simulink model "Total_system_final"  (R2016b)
settings: Solver=VariableStepAuto  StartTime=0  StopTime=2700  MaxStep=0.1  RelTol=1e-3
undefined symbols (not defined in the file or in its folder): c1, c2, c3, c4, c5, c6, cp_nom, Generation, lambda_nom, P_wind_base, Pelec_base, Pnom, re_lib, speed_nom, Turbine, Wind, wind_base
libraries: simulink x15, simulink_extras x8, dspsigops x7, realtime_pacer_lib x2

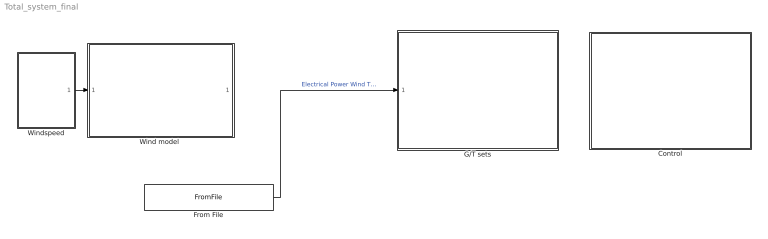
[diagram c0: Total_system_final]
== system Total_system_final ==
  Control : Subsystem
  From File : FromFile  FileName=Pwt_moderate_windtest_6mw_pu  SampleTime=0
  G/T sets : Subsystem
  "Wind model " : Subsystem  Commented=on
  Windspeed : Subsystem
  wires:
  From File/1 -> G/T sets/1(Pe_wind)  "Electrical Power Wind Turbine"
  Windspeed/1(Windspeed) -> "Wind model "/1("windspeed ")

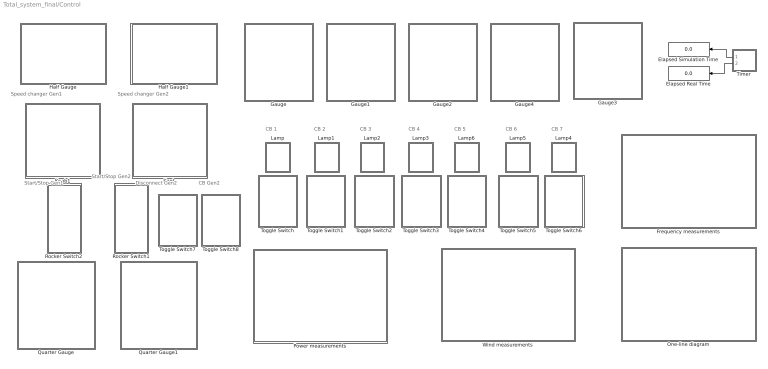
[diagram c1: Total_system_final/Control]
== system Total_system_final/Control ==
  note: Start/Stop Gen1
  note: CB 1
  note: CB 2
  note: CB 3
  note: CB 4
  note: CB 5
  note: CB 6
  note: CB 7
  note: Start/Stop Gen2
  note: Speed changer Gen2
  note: Speed changer Gen1
  note: Disconnect Gen2
  note: CB Gen2
  Elapsed Real Time : Display
  Elapsed Simulation Time : Display
  Frequency measurements : Subsystem
  Gauge : Subsystem  DialogController=hmiCreateDDGDialog  IsWebBlock=on
  Gauge1 : Subsystem  DialogController=hmiCreateDDGDialog  IsWebBlock=on
  Gauge2 : Subsystem  DialogController=hmiCreateDDGDialog  IsWebBlock=on
  Gauge3 : Subsystem  DialogController=hmiCreateDDGDialog  IsWebBlock=on
  Gauge4 : Subsystem  DialogController=hmiCreateDDGDialog  IsWebBlock=on
  Half Gauge : Subsystem  DialogController=hmiCreateDDGDialog  IsWebBlock=on
  Half Gauge1 : Subsystem  DialogController=hmiCreateDDGDialog  IsWebBlock=on
  Knob : Subsystem  DialogController=hmiCreateDDGDialog  IsWebBlock=on
  Knob1 : Subsystem  DialogController=hmiCreateDDGDialog  IsWebBlock=on
  Lamp : Subsystem  Tag=CB1  DialogController=hmiCreateDDGDialog  IsWebBlock=on
  Lamp1 : Subsystem  DialogController=hmiCreateDDGDialog  IsWebBlock=on
  Lamp2 : Subsystem  DialogController=hmiCreateDDGDialog  IsWebBlock=on
  Lamp3 : Subsystem  DialogController=hmiCreateDDGDialog  IsWebBlock=on
  Lamp4 : Subsystem  DialogController=hmiCreateDDGDialog  IsWebBlock=on
  Lamp5 : Subsystem  DialogController=hmiCreateDDGDialog  IsWebBlock=on
  Lamp6 : Subsystem  DialogController=hmiCreateDDGDialog  IsWebBlock=on
  One-line diagram : Subsystem
  Power measurements : Subsystem
  Quarter Gauge : Subsystem  DialogController=hmiCreateDDGDialog  IsWebBlock=on
  Quarter Gauge1 : Subsystem  DialogController=hmiCreateDDGDialog  IsWebBlock=on
  Rocker Switch1 : Subsystem  DialogController=hmiCreateDDGDialog  IsWebBlock=on
  Rocker Switch2 : Subsystem  DialogController=hmiCreateDDGDialog  IsWebBlock=on
  Timer : Subsystem
  Toggle Switch : Subsystem  DialogController=hmiCreateDDGDialog  IsWebBlock=on
  Toggle Switch1 : Subsystem  DialogController=hmiCreateDDGDialog  IsWebBlock=on
  Toggle Switch2 : Subsystem  DialogController=hmiCreateDDGDialog  IsWebBlock=on
  Toggle Switch3 : Subsystem  DialogController=hmiCreateDDGDialog  IsWebBlock=on
  Toggle Switch4 : Subsystem  DialogController=hmiCreateDDGDialog  IsWebBlock=on
  Toggle Switch5 : Subsystem  DialogController=hmiCreateDDGDialog  IsWebBlock=on
  Toggle Switch6 : Subsystem  DialogController=hmiCreateDDGDialog  IsWebBlock=on
  Toggle Switch7 : Subsystem  DialogController=hmiCreateDDGDialog  IsWebBlock=on
  Toggle Switch8 : Subsystem  DialogController=hmiCreateDDGDialog  IsWebBlock=on
  Wind measurements : Subsystem
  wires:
  Timer/2(Out2) -> Elapsed Real Time/1
  Timer/1(Out1) -> Elapsed Simulation Time/1

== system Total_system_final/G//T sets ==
  Pe_wind : Inport
  G/T sets : Subsystem
  Load : Subsystem
  Load shedding : Subsystem
  Mux : Mux  Inputs=2
  Scope : Scope
  Scope1 : Scope
  Start & Stop : Subsystem
  Switches : Subsystem
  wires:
  Mux/1 -> Scope/1
  G/T sets/1(Gen1freq) -> Scope1/1, Mux/1  "Frequency Gen 1"
  G/T sets/2(Gen2Freq) -> Mux/2  "Frequency Gen 2"
  Pe_wind/1 -> Load/1(Pe_wind)
  Load/1(Pe_Gen) -> Start & Stop/1(Pe_Gen), G/T sets/2(Last)
  Switches/2(Disc_Gen_2) -> G/T sets/6(Disc)
  Switches/3(Auto) -> G/T sets/1(auto), Start & Stop/3(Auto)
  Switches/6(StartStopp_Gen1) -> Start & Stop/4(StartStop_Gen1)
  Switches/7(StartStopp_Gen2) -> Start & Stop/5(StartStop_Gen2)
  Switches/4(SpeedChanger1) -> G/T sets/4(speedchanger1)
  Switches/5(SpeedChanger2) -> G/T sets/5(speedchanger2)
  Switches/1(CB_Man) -> G/T sets/3(CB_man), Start & Stop/2(CB_man)

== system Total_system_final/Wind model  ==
  "windspeed " : Inport
  Drive train model : Subsystem
  Mux : Mux  Inputs=2
  Pitch : Subsystem
  Scope : Scope
  Scope1 : Scope
  To File : ToFile  Commented=on  Filename=Pwt_moderate_windtest_6MW.mat  MatrixName=Pwt_moderate_windtest_6MW  SaveFormat=Timeseries
  Wind Turbine : Subsystem  AncestorBlock=re_lib/Wind Generation/Wind Turbine  DialogController=POWERSYS.PowerSysDialog
  Pe : Outport
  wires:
  Drive train model/1(w) -> Scope/1, Wind Turbine/1(Generator speed (pu))
  Wind Turbine/1(Tm (pu)) -> Pitch/1(Tm), Drive train model/1(Tm), Mux/1
  "windspeed "/1 -> Wind Turbine/3(Wind speed (m/s)), Pitch/2(windspeed)
  Pitch/1(ß) -> Wind Turbine/2(Pitch angle (deg))
  Mux/1 -> Scope1/1
  Drive train model/2(Pe_ref) -> To File/1, Pe/1, Mux/2

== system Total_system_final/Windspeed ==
  From File1 : FromFile  FileName=wind_forecast2.mat  SampleTime=0
  From File3 : FromFile  FileName=windserie_test.mat  SampleTime=0
  Mux : Mux  Inputs=2
  Scope : Scope
  Scope1 : Scope
  Scope2 : Scope
  Windspeed : Outport
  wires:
  From File1/1 -> Mux/1, Scope/1  "Wind forecast"
  From File3/1 -> Mux/2, Scope1/1, Windspeed/1  "Wind speed m/s"
  Mux/1 -> Scope2/1

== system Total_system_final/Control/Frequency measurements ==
  Dashboard Scope : Subsystem  DialogController=hmiCreateDDGDialog  IsWebBlock=on
  Dashboard Scope1 : Subsystem  DialogController=hmiCreateDDGDialog  IsWebBlock=on

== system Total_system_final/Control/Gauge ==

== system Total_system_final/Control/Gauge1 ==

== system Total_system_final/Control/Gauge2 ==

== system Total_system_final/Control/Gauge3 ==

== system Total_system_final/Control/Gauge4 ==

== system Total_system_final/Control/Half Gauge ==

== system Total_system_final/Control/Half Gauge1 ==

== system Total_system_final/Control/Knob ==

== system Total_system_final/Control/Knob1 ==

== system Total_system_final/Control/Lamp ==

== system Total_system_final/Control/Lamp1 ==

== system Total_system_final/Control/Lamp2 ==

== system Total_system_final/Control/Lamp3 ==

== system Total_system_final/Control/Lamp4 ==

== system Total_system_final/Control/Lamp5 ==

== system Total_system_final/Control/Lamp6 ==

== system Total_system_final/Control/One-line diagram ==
  MultiStateImage : Subsystem  DialogController=hmiCreateDDGDialog  IsWebBlock=on

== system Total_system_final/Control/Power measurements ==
  Dashboard Scope : Subsystem  DialogController=hmiCreateDDGDialog  IsWebBlock=on
  Dashboard Scope1 : Subsystem  DialogController=hmiCreateDDGDialog  IsWebBlock=on
  Dashboard Scope2 : Subsystem  DialogController=hmiCreateDDGDialog  IsWebBlock=on
  Dashboard Scope3 : Subsystem  DialogController=hmiCreateDDGDialog  IsWebBlock=on

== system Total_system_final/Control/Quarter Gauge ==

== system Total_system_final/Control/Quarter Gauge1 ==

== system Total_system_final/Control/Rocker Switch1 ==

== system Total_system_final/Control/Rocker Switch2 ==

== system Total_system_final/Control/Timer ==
  Clock : Clock
  Elapsed Real Time1 : realtime_pacer_lib/Elapsed Real Time
  Real-Time Pacer : realtime_pacer_lib/Real-Time Pacer  simTimePerRealTime=15
  Scope5 : Scope
  Subtract : Sum  Inputs=+-
  Out1 : Outport
  Out2 : Outport  Port=2
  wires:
  Clock/1 -> Out1/1, Subtract/1
  Subtract/1 -> Scope5/1  "Simulated - Real Time (seconds)"
  Elapsed Real Time1/1 -> Out2/1, Subtract/2

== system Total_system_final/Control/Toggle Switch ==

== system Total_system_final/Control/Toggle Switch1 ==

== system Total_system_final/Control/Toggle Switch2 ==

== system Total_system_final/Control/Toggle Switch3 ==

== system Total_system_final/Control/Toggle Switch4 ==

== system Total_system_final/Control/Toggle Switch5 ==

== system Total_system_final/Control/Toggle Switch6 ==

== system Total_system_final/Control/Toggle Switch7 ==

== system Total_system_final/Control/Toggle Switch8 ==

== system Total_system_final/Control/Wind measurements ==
  Dashboard Scope : Subsystem  DialogController=hmiCreateDDGDialog  IsWebBlock=on
  Dashboard Scope1 : Subsystem  DialogController=hmiCreateDDGDialog  IsWebBlock=on

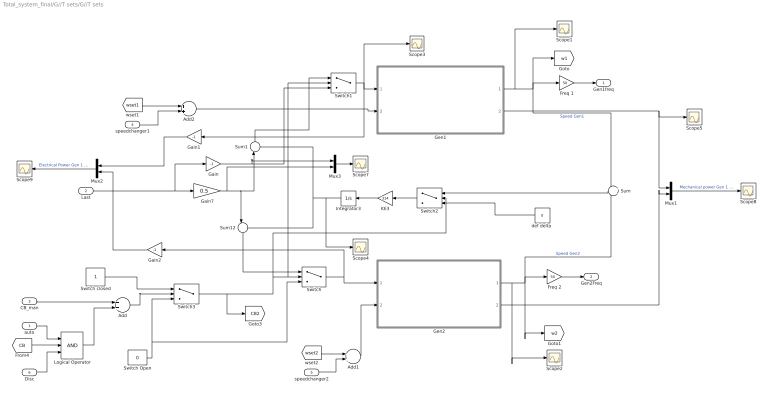
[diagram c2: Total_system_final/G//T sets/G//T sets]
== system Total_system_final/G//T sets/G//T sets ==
  auto : Inport
  Last : Inport  Port=2
  CB_man : Inport  Port=3
  speedchanger1 : Inport  Port=4
  speedchanger2 : Inport  Port=5
  Disc : Inport  Port=6
  Add : Sum
  Add1 : Sum
  Add2 : Sum
  Freq 1 : Gain  Gain=50
  Freq 2 : Gain  Gain=50
  Gain : Gain  Gain=-1
  Gain1 : Gain  Gain=-1
  Gain2 : Gain  Gain=-1
  Gain7 : Gain  Gain=0.5
  Gen1 : Subsystem
  Gen2 : Subsystem
  Integrator3 : Integrator  UpperSaturationLimit=0.0001  LowerSaturationLimit=-0.0001
  KE3 : Gain  Gain=314
  Logical Operator : Logic  Inputs=3  AllPortsSameDT=off  OutDataTypeStr=boolean
  Mux1 : Mux  Inputs=2
  Mux2 : Mux  Inputs=2
  Mux3 : Mux  Inputs=2
  Scope{1..5,7..9} (8 alike) : Scope
  Sum : Sum  Inputs=+-
  Sum1 : Sum  Inputs=--
  Sum12 : Sum  Inputs=|-+
  Switch{,1..3} (4 alike) : Switch  Criteria=u2 > Threshold
  Switch Open : Constant  Value=0
  Switch closed : Constant
  "def delta " : Constant  Value=0
  Gen1freq : Outport
  Gen2Freq : Outport  Port=2
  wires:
  Gen2/1(w2) -> Scope2/1, [w2], Sum/2, Freq 2/1  "Speed Gen2"
  Gen1/1(w1) -> Scope1/1, [w1], Sum/1, Freq 1/1  "Speed Gen1"
  Mux1/1 -> Scope8/1  "Mechanical power Gen 1 and 2"
  Gen1/2(Pm1) -> Scope5/1, Mux1/1
  Gen2/2(Pm2) -> Mux1/2
  Mux2/1 -> Scope9/1  "Electrical Power Gen 1 & 2"
  Gain7/1 -> Mux3/2, Sum1/1, Sum12/1
  Switch2/1 -> KE3/1
  Switch1/1 -> Scope3/1, Gain1/1, Gen1/1(Pe)
  Sum1/1 -> Switch1/1
  Switch/1 -> Gen2/1(Pe), Gain2/1
  Sum12/1 -> Switch/1
  Switch3/1 -> [CB2], Switch2/2, Switch1/2, Switch/2
  Switch Open/1 -> Switch/3, Switch3/3
  Switch closed/1 -> Switch3/1
  Gain/1 -> Mux3/1, Switch1/3
  Integrator3/1 -> Scope4/1, Sum1/2, Sum12/2
  KE3/1 -> Integrator3/1
  "def delta "/1 -> Switch2/3
  Freq 1/1 -> Gen1freq/1
  Freq 2/1 -> Gen2Freq/1
  Mux3/1 -> Scope7/1
  speedchanger1/1 -> Add2/2
  [wset1] -> Add2/1
  Add2/1 -> Gen1/2(wset1)
  Add/1 -> Switch3/2
  Last/1 -> Gain/1, Gain7/1
  Add1/1 -> Gen2/2(wset2)
  speedchanger2/1 -> Add1/2
  Logical Operator/1 -> Add/2
  [CB] -> Logical Operator/2
  auto/1 -> Logical Operator/1
  CB_man/1 -> Add/1
  Disc/1 -> Logical Operator/3
  Gain1/1 -> Mux2/1
  Gain2/1 -> Mux2/2
  Sum/1 -> Switch2/1
  [wset2] -> Add1/1

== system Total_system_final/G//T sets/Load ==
  Pe_wind : Inport
  Add : Sum  Inputs=+-
  Local base --> System base : Gain  Gain=6/13
  Pe_Gen : Outport
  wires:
  Add/1 -> Pe_Gen/1
  Local base --> System base/1 -> Add/2, [P_wind]  "Electrical Power Wind turbine"
  [Pe_load] -> Add/1  "Electrical load"
  Pe_wind/1 -> Local base --> System base/1

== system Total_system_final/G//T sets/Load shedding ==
  Display{,1..3,5..8} (8 alike) : Display
  Load shedding : Subsystem
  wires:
  Load shedding/2(Open CB_B1M1) -> Display/1
  Load shedding/1(∆Pe_G1) -> [Pe_load]
  Load shedding/3(Open CB_B1M2) -> Display1/1
  Load shedding/4(Open CB_B1L1) -> Display2/1
  Load shedding/5(Open CB_B1M3) -> Display3/1
  [w1] -> Load shedding/1(w_G1)
  Load shedding/7(Open CB_B1B4) -> Display6/1
  Load shedding/6(Open CB_B1M4) -> Display5/1
  Load shedding/8(Open CB_B4B5) -> Display7/1
  Load shedding/9(idx) -> Display8/1

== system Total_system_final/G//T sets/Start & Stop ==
  Pe_Gen : Inport
  CB_man : Inport  Port=2
  Auto : Inport  Port=3
  StartStop_Gen1 : Inport  Port=4
  StartStop_Gen2 : Inport  Port=5
  StartStop : MATLAB Function  TreatAsAtomicUnit=on
  TransportDelay : TransportDelay  DelayTime=400
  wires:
  Pe_Gen/1 -> StartStop/1(P_Gen)
  CB_man/1 -> StartStop/2(CB_man)
  Auto/1 -> StartStop/7(auto)
  StartStop/2(wset2) -> [wset2]
  StartStop/3(CB_auto) -> TransportDelay/1
  [w2] -> StartStop/4(w2)
  TransportDelay/1 -> StartStop/8(Connect), [CB]
  [w1] -> StartStop/3(w1)
  StartStop/1(wset1) -> [wset1]
  StartStop_Gen1/1 -> StartStop/5(start_stop_G1)
  StartStop_Gen2/1 -> StartStop/6(start_stop_G2)

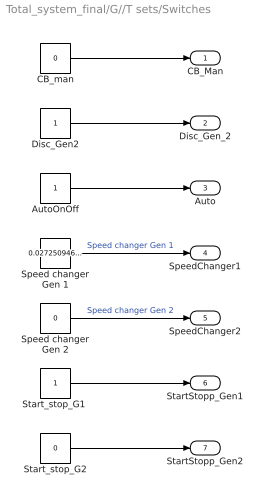
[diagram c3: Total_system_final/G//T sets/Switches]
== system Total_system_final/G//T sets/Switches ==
  AutoOnOff : Constant
  CB_man : Constant  Value=0
  Disc_Gen2 : Constant
  Speed changer Gen 1 : Constant  Value=0.0272509460449
  Speed changer Gen 2 : Constant  Value=0
  "Start_stop_G1 " : Constant
  Start_stop_G2 : Constant  Value=0
  CB_Man : Outport
  Disc_Gen_2 : Outport  Port=2
  Auto : Outport  Port=3
  SpeedChanger1 : Outport  Port=4
  SpeedChanger2 : Outport  Port=5
  StartStopp_Gen1 : Outport  Port=6
  StartStopp_Gen2 : Outport  Port=7
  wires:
  "Start_stop_G1 "/1 -> StartStopp_Gen1/1
  AutoOnOff/1 -> Auto/1
  Disc_Gen2/1 -> Disc_Gen_2/1
  CB_man/1 -> CB_Man/1
  Speed changer Gen 1/1 -> SpeedChanger1/1  "Speed changer Gen 1"
  Speed changer Gen 2/1 -> SpeedChanger2/1  "Speed changer Gen 2"
  Start_stop_G2/1 -> StartStopp_Gen2/1

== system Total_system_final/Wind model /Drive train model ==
  Tm : Inport
  Controller : Subsystem
  Gain : Gain  Gain=1/(2*5)
  Integrator : Integrator  InitialCondition=1  LimitOutput=on  UpperSaturationLimit=2  LowerSaturationLimit=0
  Sum : Sum  Inputs=|+|-
  Transfer Fcn : TransferFcn  Denominator=[2 1]
  w : Outport
  Pe_ref : Outport  Port=2
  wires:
  Tm/1 -> Sum/1
  Sum/1 -> Gain/1
  Gain/1 -> Integrator/1
  Integrator/1 -> Controller/1(In1), w/1
  Transfer Fcn/1 -> Pe_ref/1, Sum/2
  Controller/1(Out1) -> Transfer Fcn/1

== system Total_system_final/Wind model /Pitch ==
  Tm : Inport
  windspeed : Inport  Port=2
  Delay : TransferFcn  Denominator=[0.1 1]
  Integrator Limited : Integrator  LimitOutput=on  UpperSaturationLimit=90  LowerSaturationLimit=0
  PI : Subsystem
  Rate Limiter : RateLimiter  RisingSlewLimit=5  FallingSlewLimit=-5
  Saturation2 : Saturate  UpperLimit=90  LowerLimit=0  ZeroCross=off
  Saturation3 : Saturate  UpperLimit=1  LowerLimit=-1  ZeroCross=off
  Sum1 : Sum  Inputs=|+|-
  Sum2 : Sum  Inputs=|+-
  Tm_ref : Constant
  ß : Outport
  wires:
  Tm_ref/1 -> Sum1/2
  Delay/1 -> Rate Limiter/1
  Rate Limiter/1 -> Integrator Limited/1
  windspeed/1 -> PI/2(Wind speed)
  Saturation3/1 -> PI/1(∆Tm)
  PI/1(Out1) -> Saturation2/1
  Sum2/1 -> Delay/1
  Saturation2/1 -> Sum2/1
  Sum1/1 -> Saturation3/1
  Tm/1 -> Sum1/1
  Integrator Limited/1 -> Sum2/2, ß/1

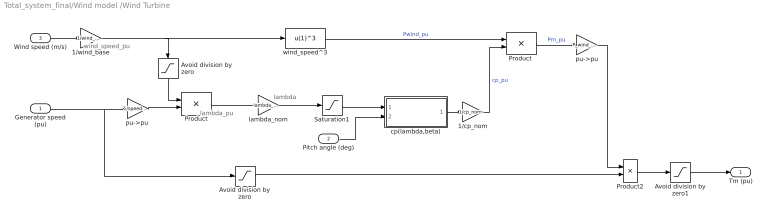
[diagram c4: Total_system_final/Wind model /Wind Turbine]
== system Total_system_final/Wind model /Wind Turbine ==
  note: wind_speed_pu
  note: lambda_pu
  note: lambda
  Generator speed (pu) : Inport
  Pitch angle (deg) : Inport  Port=2
  Wind speed (m/s) : Inport  Port=3
  1/cp_nom : Gain  Gain=1/cp_nom
  1/wind_base : Gain  Gain=1/wind_base
  Avoid division by zero : Saturate  UpperLimit=1e6  LowerLimit=1e-6
  "Avoid division by zero " : Saturate  UpperLimit=1e6  LowerLimit=1e-6
  Avoid division by zero1 : Saturate  UpperLimit=3  LowerLimit=0
  Product : Product  Inputs=/*
  "Product " : Product
  Product2 : Product  Inputs=*/
  Saturation1 : Saturate  UpperLimit=inf  LowerLimit=1e-6
  cp(lambda,beta) : Subsystem
  lambda_nom : Gain  Gain=lambda_nom
  pu->pu : Gain  Gain=P_wind_base*Pnom/Pelec_base
  "pu->pu " : Gain  Gain=1/speed_nom
  wind_speed^3 : Fcn  Expr=u(1)^3
  Tm (pu) : Outport
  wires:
  Pitch angle (deg)/1 -> cp(lambda,beta)/2(beta)
  pu->pu/1 -> Product2/1
  cp(lambda,beta)/1(cp) -> 1/cp_nom/1
  wind_speed^3/1 -> "Product "/1  "Pwind_pu"
  Avoid division by zero/1 -> Product2/2
  Wind speed (m/s)/1 -> 1/wind_base/1
  Generator speed (pu)/1 -> Avoid division by zero/1, "pu->pu "/1
  "Product "/1 -> pu->pu/1  "Pm_pu"
  lambda_nom/1 -> Saturation1/1
  1/cp_nom/1 -> "Product "/2  "cp_pu"
  Saturation1/1 -> cp(lambda,beta)/1(lambda)
  Product/1 -> lambda_nom/1
  1/wind_base/1 -> wind_speed^3/1, "Avoid division by zero "/1
  "Avoid division by zero "/1 -> Product/1
  "pu->pu "/1 -> Product/2
  Product2/1 -> Avoid division by zero1/1
  Avoid division by zero1/1 -> Tm (pu)/1

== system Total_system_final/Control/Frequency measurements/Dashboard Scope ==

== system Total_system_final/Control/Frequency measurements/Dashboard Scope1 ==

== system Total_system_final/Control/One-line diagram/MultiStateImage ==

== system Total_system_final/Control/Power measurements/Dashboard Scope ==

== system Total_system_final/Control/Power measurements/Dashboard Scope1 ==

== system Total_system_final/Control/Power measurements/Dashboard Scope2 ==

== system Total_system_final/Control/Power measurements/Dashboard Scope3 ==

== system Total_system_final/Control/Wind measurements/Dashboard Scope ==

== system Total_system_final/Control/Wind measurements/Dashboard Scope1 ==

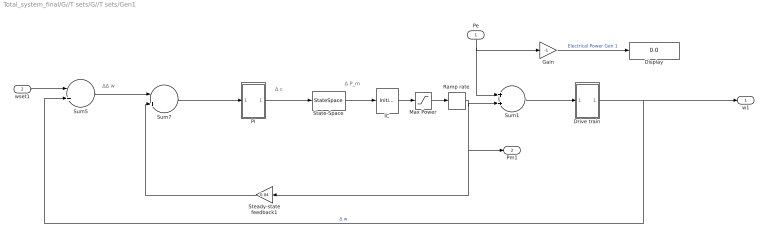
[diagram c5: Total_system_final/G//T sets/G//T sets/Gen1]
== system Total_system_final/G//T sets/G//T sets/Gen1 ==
  note: ∆∆ w
  note: ∆ c
  note: ∆ P_m
  Pe : Inport
  wset1 : Inport  Port=2
  Display : Display
  Drive train : Subsystem
  Gain : Gain  Gain=-1
  IC : InitialCondition
  Max Power : Saturate  Commented=through  UpperLimit=1.2  LowerLimit=-0.2
  PI : Subsystem
  Ramp rate : RateLimiter  Commented=through  RisingSlewLimit=0.05  SampleTimeMode=inherited
  State-Space : StateSpace  A=-5  C=5  D=0  X0=0
  Steady-state feedback1 : Gain  Gain=0.04
  Sum1 : Sum
  Sum5 : Sum  Inputs=|+|-
  Sum7 : Sum  Inputs=|+|-
  w1 : Outport
  Pm1 : Outport  Port=2
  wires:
  Pe/1 -> Sum1/1, Gain/1
  Sum5/1 -> Sum7/1
  Steady-state feedback1/1 -> Sum7/2
  Sum7/1 -> PI/1(In1)
  Sum1/1 -> Drive train/1(In1)
  wset1/1 -> Sum5/1
  Drive train/1(Out1) -> w1/1, Sum5/2  "∆ w"
  PI/1(Out1) -> State-Space/1
  Gain/1 -> Display/1  "Electrical Power Gen 1"
  Max Power/1 -> Ramp rate/1
  Ramp rate/1 -> Steady-state feedback1/1, Pm1/1, Sum1/2
  State-Space/1 -> IC/1
  IC/1 -> Max Power/1

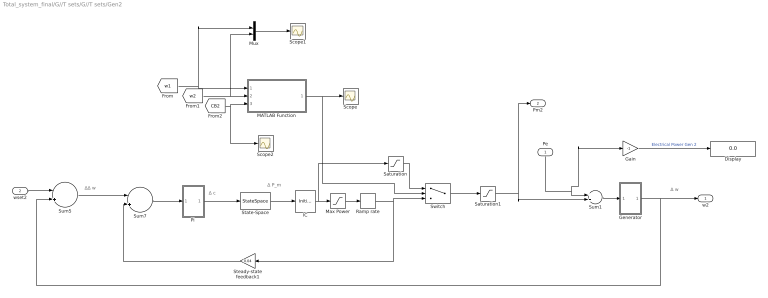
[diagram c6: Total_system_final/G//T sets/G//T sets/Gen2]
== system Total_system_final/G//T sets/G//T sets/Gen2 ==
  note: ∆∆ w
  note: ∆ w
  note: ∆ c
  note: ∆ P_m
  Pe : Inport
  wset2 : Inport  Port=2
  Display : Display
  Gain : Gain  Gain=-1
  Generator : Subsystem
  IC : InitialCondition  Commented=through
  MATLAB Function : MATLAB Function  TreatAsAtomicUnit=on
  Max Power : Saturate  Commented=through  UpperLimit=1.05  LowerLimit=-0.2
  Mux : Mux  Inputs=2
  Pi : Subsystem
  Ramp rate : RateLimiter  Commented=through  RisingSlewLimit=0.038  SampleTimeMode=inherited
  Saturation : Saturate  UpperLimit=0.05  LowerLimit=-0.1  LinearizeAsGain=off
  Saturation1 : Saturate  UpperLimit=1.05  LowerLimit=-0.2
  Scope : Scope
  Scope1 : Scope
  Scope2 : Scope
  State-Space : StateSpace  A=-5  C=5  D=0  X0=0
  Steady-state feedback1 : Gain  Gain=0.04
  Sum1 : Sum
  Sum5 : Sum  Inputs=|+|-
  Sum7 : Sum  Inputs=|+|-
  Switch : Switch  Criteria=u2 > Threshold
  w2 : Outport
  Pm2 : Outport  Port=2
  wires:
  Sum5/1 -> Sum7/1
  Steady-state feedback1/1 -> Sum7/2
  wset2/1 -> Sum5/1
  Sum1/1 -> Generator/1(In1)
  Generator/1(Out1) -> w2/1, Sum5/2
  Sum7/1 -> Pi/1(In1)
  [w1] -> Mux/1, MATLAB Function/1(w1)
  [w2] -> Mux/2, MATLAB Function/2(w2)
  Pi/1(Out1) -> State-Space/1
  Saturation/1 -> Switch/1
  MATLAB Function/1(x) -> Switch/2, Scope/1
  [CB2] -> Scope2/1, MATLAB Function/3(CB)
  Pe/1 -> Gain/1, Sum1/1
  Gain/1 -> Display/1  "Electrical Power Gen 2"
  Mux/1 -> Scope1/1
  Saturation1/1 -> Sum1/2, Pm2/1
  Switch/1 -> Saturation1/1
  Max Power/1 -> Ramp rate/1
  IC/1 -> Saturation/1, Max Power/1
  State-Space/1 -> IC/1
  Ramp rate/1 -> Steady-state feedback1/1, Switch/3

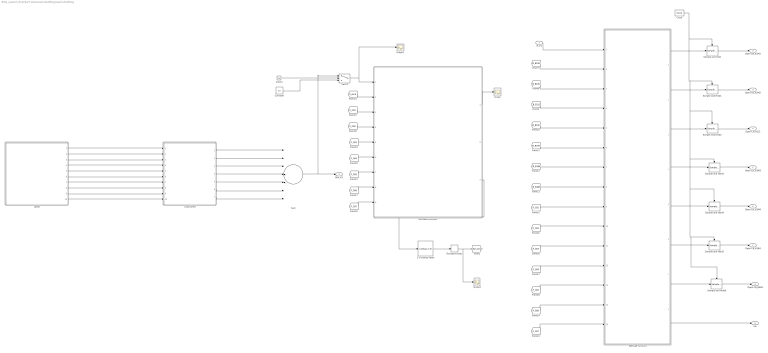
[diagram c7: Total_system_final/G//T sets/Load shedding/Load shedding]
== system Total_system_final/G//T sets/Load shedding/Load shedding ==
  w_G1 : Inport
  1-D Lookup Table : Lookup_n-D  NumberOfTableDimensions=1  BreakpointsForDimension1=[0,1,2,3,4,5,6,7]  Table=[0 10, 12, 14, 16, 18, 20, 22]  InternalRulePriority=Speed  RndMeth=Simplest
  Clock : simulink_extras/Flip Flops/Clock  period=10
  Clock1 : Clock
  Constant : Constant  Value=0.8
  Load_Shed : Subsystem
  Loads : Subsystem
  MATLAB Function : MATLAB Function  TreatAsAtomicUnit=on
  MATLAB Function1 : MATLAB Function  TreatAsAtomicUnit=on
  Sample and Hold{,1..6} (7 alike) : dspsigops/Sample and Hold  trig=Rising edge  initCond=0  latchinput=off
  Scope : Scope
  Scope1 : Scope
  Scope2 : Scope
  Sum : Sum  Inputs=+++++++
  Switch : Switch  Criteria=u2 > Threshold  Threshold=199
  Transport Delay : TransportDelay
  ∆Pe_G1 : Outport
  Open CB_B1M1 : Outport  Port=2
  Open CB_B1M2 : Outport  Port=3
  Open CB_B1L1 : Outport  Port=4
  Open CB_B1M3 : Outport  Port=5
  Open CB_B1M4 : Outport  Port=6
  Open CB_B1B4 : Outport  Port=7
  Open CB_B4B5 : Outport  Port=8
  idx : Outport  Port=9
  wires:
  w_G1/1 -> MATLAB Function/1(freq)
  Loads/1("Load M1 ") -> Load_Shed/1(" Load M1")
  Loads/10(Load M7) -> Load_Shed/10(Load M7)
  Loads/9(Load L3) -> Load_Shed/9(Load L3)
  Loads/8(Load M6) -> Load_Shed/8(Load M6)
  Loads/7(Load M5) -> Load_Shed/7(Load M5)
  Loads/6(Load L2) -> Load_Shed/6(Load L2)
  Loads/5(Load M4) -> Load_Shed/5(Load M4)
  Loads/4(Load M3) -> Load_Shed/4(Load M3)
  Loads/3(Load L1) -> Load_Shed/3(Load L1)
  Loads/2(Load M2) -> Load_Shed/2(Load M2)
  [CB_B1M1] -> MATLAB Function/2(CB_B1M1)
  [CB_B1M2] -> MATLAB Function/3(CB_B1M2)
  [CB_B1L1] -> MATLAB Function/4(CB_B1L1)
  [CB_B1M3] -> MATLAB Function/5(CB_B1M3)
  [CB_B1M4] -> MATLAB Function/6(CB_B1M4)
  [CB_B1B4] -> MATLAB Function/7(CB_B1B4)
  [CB_B4B5] -> MATLAB Function/8(CB_B4B5)
  [P_CB1] -> MATLAB Function/9(P_CB_B1M1)
  [P_CB2] -> MATLAB Function/10(P_CB_B1M2)
  [P_CB3] -> MATLAB Function/11(P_CB_B1L1)
  [P_CB4] -> MATLAB Function/12(P_CB_B1M3)
  [P_CB5] -> MATLAB Function/13(P_CB_B1M4)
  [P_CB6] -> MATLAB Function/14(P_CB_B1B4)
  [P_CB7] -> MATLAB Function/15(P_CB_B4B5)
  MATLAB Function/1(CB_B1M1_stat) -> Sample and Hold/1
  Sample and Hold/1 -> Open CB_B1M1/1
  MATLAB Function/8(idx) -> idx/1
  MATLAB Function/2(CB_B1M2_stat) -> Sample and Hold1/1
  Sample and Hold1/1 -> Open CB_B1M2/1
  Sample and Hold2/1 -> Open CB_B1L1/1
  MATLAB Function/3(CB_B1L1_stat) -> Sample and Hold2/1
  Sample and Hold3/1 -> Open CB_B1M3/1
  MATLAB Function/4(CB_B1M3_stat) -> Sample and Hold3/1
  Sample and Hold4/1 -> Open CB_B1M4/1
  MATLAB Function/5(CB_B1M4_stat) -> Sample and Hold4/1
  MATLAB Function/6(CB_B1B4_stat) -> Sample and Hold5/1
  Sample and Hold5/1 -> Open CB_B1B4/1
  MATLAB Function/7(CB_B4B5_stat) -> Sample and Hold6/1
  Sample and Hold6/1 -> Open CB_B4B5/1
  Clock/1 -> Sample and Hold6/Trigger, Sample and Hold5/Trigger, Sample and Hold4/Trigger, Sample and Hold3/Trigger, Sample and Hold2/Trigger, Sample and Hold1/Trigger, Sample and Hold/Trigger
  Sum/1 -> Switch/1, ∆Pe_G1/1
  [P_wind] -> MATLAB Function1/2(P_wind)
  MATLAB Function1/1(Power) -> Scope/1
  [P_CB1] -> MATLAB Function1/3(P_CB_B1M1)
  [P_CB2] -> MATLAB Function1/4(P_CB_B1M2)
  [P_CB3] -> MATLAB Function1/5(P_CB_B1L1)
  [P_CB4] -> MATLAB Function1/6(P_CB_B1M3)
  [P_CB5] -> MATLAB Function1/7(P_CB_B1M4)
  [P_CB6] -> MATLAB Function1/8(P_CB_B1B4)
  [P_CB7] -> MATLAB Function1/9(P_CB_B4B5)
  MATLAB Function1/3(CB) -> 1-D Lookup Table/1
  1-D Lookup Table/1 -> Transport Delay/1
  Transport Delay/1 -> [CB2_auto2], Scope2/1
  Load_Shed/1(Power_CB_B1M1) -> Sum/1
  Load_Shed/2(Power_CB_B1M2) -> Sum/2
  Load_Shed/3(Power_CB_B1L1) -> Sum/3
  Load_Shed/4(Power_CB_B1M3) -> Sum/4
  Load_Shed/5(Power_CB_B1M4) -> Sum/5
  Load_Shed/6(Power_CB_B4B5) -> Sum/6
  Load_Shed/7(Power_CB_B1B4) -> Sum/7
  Switch/1 -> Scope1/1, MATLAB Function1/1(P_load)
  Clock1/1 -> Switch/2
  Constant/1 -> Switch/3

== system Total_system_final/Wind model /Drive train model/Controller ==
  In1 : Inport
  Fcn : Fcn  Expr=u^2
  "MW -> pu" : Gain  Gain=1/(6e6)
  Product : Product
  Subsystem : Subsystem
  "pu -> rad/sec" : Gain  Gain=11*((2*3.14)/60)
  Out1 : Outport
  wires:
  Product/1 -> "MW -> pu"/1
  Fcn/1 -> Product/1
  Subsystem/1(K-opt) -> Product/2
  "pu -> rad/sec"/1 -> Fcn/1
  In1/1 -> "pu -> rad/sec"/1
  "MW -> pu"/1 -> Out1/1

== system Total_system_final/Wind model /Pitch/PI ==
  ∆Tm : Inport
  Wind speed : Inport  Port=2
  Gain scheduling : Lookup_n-D  NumberOfTableDimensions=1  BreakpointsForDimension1=[10,12,14,15,16,17,18,19,20,21,22,23,24,25]  Table=[20,20,20,20,20,20,20,20,15,15,15,15,15,15]  InternalRulePriority=Speed  RndMeth=Simplest
  Integral constant : Constant  Value=3.11111
  PI Controller : simulink/Continuous/PID Controller  Controller=PI  TimeDomain=Continuous-time  SampleTime=-1  IntegratorMethod=Forward Euler  FilterMethod=Forward Euler  Form=Parallel  UseFilter=on  ControllerParametersSource=external  P=1  I=1  D=0  N=100  InitialConditionSource=internal  InitialConditionForIntegrator=0  InitialConditionForFilter=0  ExternalReset=none  LimitOutput=on  UpperSaturationLimit=90  LowerSaturationLimit=0  LinearizeAsGain=on  AntiWindupMode=clamping  Kb=1  TrackingMode=off  Kt=1  PParamMin=[]  PParamMax=[]  IParamMin=[]  IParamMax=[]  DParamMin=[]  DParamMax=[]  NParamMin=[]  NParamMax=[]  KbParamMin=[]  KbParamMax=[]  KtParamMin=[]  KtParamMax=[]  POutMin=[]  POutMax=[]  IOutMin=[0]  IOutMax=[]  DOutMin=[]  DOutMax=[]  NOutMin=[]  NOutMax=[]  KbOutMin=[]  KbOutMax=[]  KtOutMin=[]  KtOutMax=[]  IntegratorOutMin=[]  IntegratorOutMax=[]  FilterOutMin=[]  FilterOutMax=[]  SumOutMin=[]  SumOutMax=[]  SumI1OutMin=[]  SumI1OutMax=[]  SumI2OutMin=[]  SumI2OutMax=[]  SumI3OutMin=[]  SumI3OutMax=[]  SumDOutMin=[]  SumDOutMax=[]  SaturationOutMin=[]  SaturationOutMax=[]  IntegratorContinuousStateAttributes=''  IntegratorStateMustResolveToSignalObject=off  IntegratorRTWStateStorageClass=Auto  FilterContinuousStateAttributes=''  FilterStateMustResolveToSignalObject=off  FilterRTWStateStorageClass=Auto  DifferentiatorICPrevScaledInput=0  DifferentiatorOutMin=[]  DifferentiatorOutMax=[]
  Out1 : Outport
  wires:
  Gain scheduling/1 -> PI Controller/2
  Wind speed/1 -> Gain scheduling/1
  ∆Tm/1 -> PI Controller/1
  PI Controller/1 -> Out1/1
  Integral constant/1 -> PI Controller/3

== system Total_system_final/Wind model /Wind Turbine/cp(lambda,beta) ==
  lambda : Inport
  beta : Inport  Port=2
  Fcn : Fcn  Expr=1/(1/(u[1]+0.08*u[2])-0.035/(u[2]^3+1))
  Fcn1 : Fcn  Expr=c1*(c2/u[2]-c3*u[3]-c4)*exp(-c5/u[2])+c6*u[1]
  Mux : Mux  Inputs=2
  Mux1 : Mux  Inputs=3
  Scope1 : Scope
  Scope2 : Scope  NumInputPorts=2
  Scope3 : Scope
  cp : Outport
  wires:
  Fcn/1 -> Scope1/1, Mux1/2  "lambda_i"
  Fcn1/1 -> Scope3/1, cp/1
  lambda/1 -> Scope2/1, Mux1/1, Mux/1
  Mux1/1 -> Fcn1/1
  beta/1 -> Scope2/2, Mux1/3, Mux/2
  Mux/1 -> Fcn/1

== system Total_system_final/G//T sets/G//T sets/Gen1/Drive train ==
  In1 : Inport
  " D" : Gain  Gain=0
  Gain4 : Gain  Gain=1/(2*5)
  Integrator Limited1 : Integrator  InitialCondition=1  UpperSaturationLimit=2  LowerSaturationLimit=0
  Sum8 : Sum  Inputs=+-
  Out1 : Outport
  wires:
  Sum8/1 -> Gain4/1
  Gain4/1 -> Integrator Limited1/1
  In1/1 -> Sum8/1
  " D"/1 -> Sum8/2
  Integrator Limited1/1 -> " D"/1, Out1/1

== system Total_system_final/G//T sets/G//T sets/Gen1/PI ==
  In1 : Inport
  Derivative : Derivative
  Gain1 : Gain  Gain=0.8
  Gain3 : Gain  Gain=5
  Gain5 : Gain  Gain=1.2
  Integrator1 : Integrator  InitialCondition=0.5
  Sum6 : Sum  Inputs=|+|+|+
  Out1 : Outport
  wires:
  Sum6/1 -> Out1/1
  Integrator1/1 -> Sum6/2
  Gain5/1 -> Integrator1/1
  In1/1 -> Gain1/1, Gain5/1, Gain3/1
  Gain3/1 -> Sum6/1
  Gain1/1 -> Derivative/1
  Derivative/1 -> Sum6/3

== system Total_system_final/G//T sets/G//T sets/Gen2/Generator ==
  In1 : Inport
  " D" : Gain  Gain=0
  Gain4 : Gain  Gain=1/(2*5)
  Integrator Limited1 : Integrator  UpperSaturationLimit=2  LowerSaturationLimit=0
  Sum8 : Sum  Inputs=+-
  Out1 : Outport
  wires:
  Sum8/1 -> Gain4/1
  Gain4/1 -> Integrator Limited1/1
  In1/1 -> Sum8/1
  " D"/1 -> Sum8/2
  Integrator Limited1/1 -> " D"/1, Out1/1

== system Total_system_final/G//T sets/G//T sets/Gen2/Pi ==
  In1 : Inport
  Derivative : Derivative
  Gain1 : Gain  Gain=0.8
  Gain3 : Gain  Gain=5
  Gain5 : Gain  Gain=1.2
  Integrator1 : Integrator  InitialCondition=0.5
  Sum6 : Sum  Inputs=|+|+|+
  Out1 : Outport
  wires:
  Sum6/1 -> Out1/1
  Integrator1/1 -> Sum6/2
  Gain5/1 -> Integrator1/1
  In1/1 -> Gain1/1, Gain5/1, Gain3/1
  Gain3/1 -> Sum6/1
  Gain1/1 -> Derivative/1
  Derivative/1 -> Sum6/3

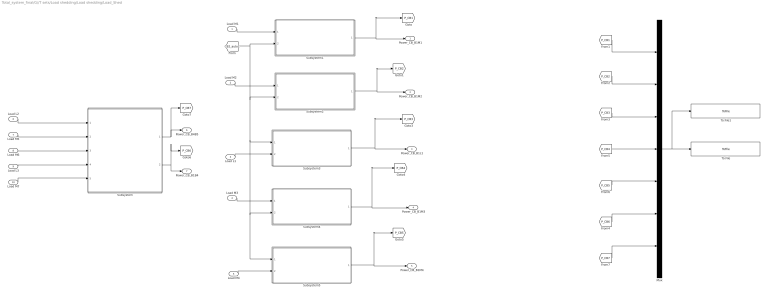
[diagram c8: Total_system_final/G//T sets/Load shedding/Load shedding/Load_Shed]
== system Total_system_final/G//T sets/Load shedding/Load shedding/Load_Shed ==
  " Load M1" : Inport
  Load M2 : Inport  Port=2
  Load L1 : Inport  Port=3
  Load M3 : Inport  Port=4
  Load M4 : Inport  Port=5
  Load L2 : Inport  Port=6
  Load M5 : Inport  Port=7
  Load M6 : Inport  Port=8
  Load L3 : Inport  Port=9
  Load M7 : Inport  Port=10
  Mux : Mux  Inputs=7
  Subsystem : Subsystem
  Subsystem1 : Subsystem
  Subsystem2 : Subsystem
  Subsystem3 : Subsystem
  Subsystem4 : Subsystem
  Subsystem5 : Subsystem
  To File : ToFile  Commented=on  Filename=Loads_Gen1_Storm_2MW.mat  MatrixName=Loads_Gen1_Storm_2MW  SaveFormat=Timeseries
  To File1 : ToFile  Commented=on  Filename=Loads_Gen1_Storm_6MW_A.mat  MatrixName=Loads_Gen1_Storm_6MW_A
  Power_CB_B1M1 : Outport
  Power_CB_B1M2 : Outport  Port=2
  Power_CB_B1L1 : Outport  Port=3
  Power_CB_B1M3 : Outport  Port=4
  Power_CB_B1M4 : Outport  Port=5
  Power_CB_B4B5 : Outport  Port=6
  Power_CB_B1B4 : Outport  Port=7
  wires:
  Load L2/1 -> Subsystem/1(Load L2)
  Load M5/1 -> Subsystem/2(Load M5)
  Load M6/1 -> Subsystem/3(Load M6)
  Load L3/1 -> Subsystem/4(Load L3)
  Load M7/1 -> Subsystem/5(Load M7)
  Subsystem/2(CB_B1B4_stat) -> [P_CB6], Power_CB_B1B4/1
  " Load M1"/1 -> Subsystem1/1(" Load M1")
  Subsystem1/1(Power_CB_B1M1) -> [P_CB1], Power_CB_B1M1/1
  [CB2_auto2] -> Subsystem1/2(In1), Subsystem5/1(In3), Subsystem4/2(In5), Subsystem3/1(In1), Subsystem2/2(In1)
  Load M2/1 -> Subsystem2/1(Load M2)
  Load L1/1 -> Subsystem3/2(Load L1)
  Subsystem2/1(Power_CB_B1M2) -> [P_CB2], Power_CB_B1M2/1
  Subsystem3/1(Power_CB_B1L1) -> [P_CB3], Power_CB_B1L1/1
  Load M3/1 -> Subsystem4/1(Load M3)
  Subsystem4/1(Power_CB_B1M3) -> [P_CB4], Power_CB_B1M3/1
  Load M4/1 -> Subsystem5/2(Load M4)
  Subsystem5/1(Power_CB_B1M4) -> [P_CB5], Power_CB_B1M4/1
  Subsystem/1(CB_B4B5_stat) -> [P_CB7], Power_CB_B4B5/1
  Mux/1 -> To File1/1, To File/1
  [P_CB1] -> Mux/1
  [P_CB3] -> Mux/3
  [P_CB2] -> Mux/2
  [P_CB4] -> Mux/4
  [P_CB5] -> Mux/5
  [P_CB6] -> Mux/6
  [P_CB7] -> Mux/7

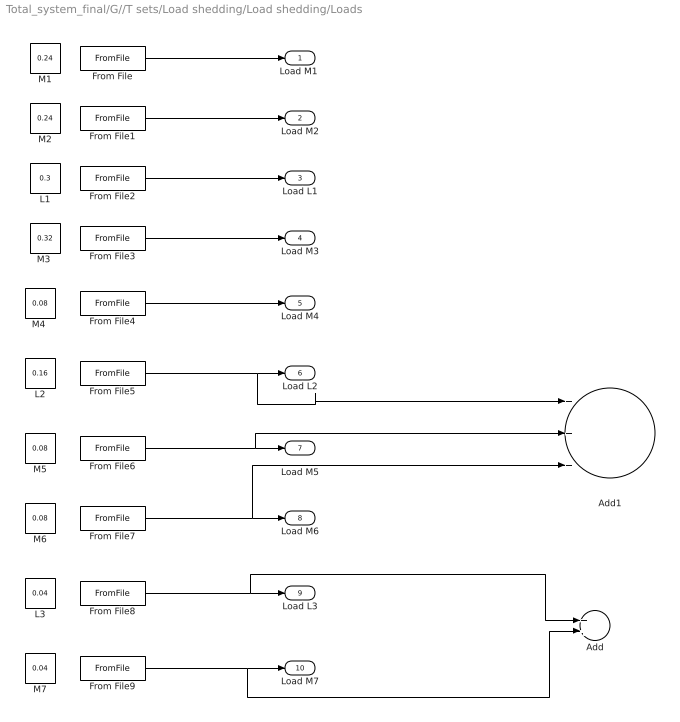
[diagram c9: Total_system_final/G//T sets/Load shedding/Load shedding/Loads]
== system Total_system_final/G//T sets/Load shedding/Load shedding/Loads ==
  Add : Sum
  Add1 : Sum  Inputs=+++
  From File : FromFile  FileName=Load_M1.mat  SampleTime=0
  From File1 : FromFile  FileName=Load_M2.mat  SampleTime=0
  From File2 : FromFile  FileName=Load_L1.mat  SampleTime=0
  From File3 : FromFile  FileName=Load_M3.mat  SampleTime=0
  From File4 : FromFile  FileName=Load_M4.mat  SampleTime=0
  From File5 : FromFile  FileName=Load_L2.mat  SampleTime=0
  From File6 : FromFile  FileName=Load_M5.mat  SampleTime=0
  From File7 : FromFile  FileName=Load_M6.mat  SampleTime=0
  From File8 : FromFile  FileName=Load_L3.mat  SampleTime=0
  From File9 : FromFile  FileName=Load_M7.mat  SampleTime=0
  L1 : Constant  Value=0.3
  L2 : Constant  Value=0.16
  L3 : Constant  Value=0.04
  M1 : Constant  Value=0.24
  M2 : Constant  Value=0.24
  "M3 " : Constant  Value=0.32
  "M4 " : Constant  Value=0.08
  M5 : Constant  Value=0.08
  M6 : Constant  Value=0.08
  M7 : Constant  Value=0.04
  "Load M1 " : Outport
  Load M2 : Outport  Port=2
  Load L1 : Outport  Port=3
  Load M3 : Outport  Port=4
  Load M4 : Outport  Port=5
  Load L2 : Outport  Port=6
  Load M5 : Outport  Port=7
  Load M6 : Outport  Port=8
  Load L3 : Outport  Port=9
  Load M7 : Outport  Port=10
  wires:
  From File/1 -> "Load M1 "/1
  From File1/1 -> Load M2/1
  From File2/1 -> Load L1/1
  From File3/1 -> Load M3/1
  From File6/1 -> Add1/2, Load M5/1
  From File7/1 -> Add1/3, Load M6/1
  From File8/1 -> Load L3/1, Add/1
  From File9/1 -> Add/2, Load M7/1
  From File5/1 -> Add1/1, Load L2/1
  From File4/1 -> Load M4/1

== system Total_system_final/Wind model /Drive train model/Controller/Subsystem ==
  Cp_max : Constant  Value=0.48
  Divide : Product  Inputs=*/
  Fcn : Fcn  Expr=u^3
  Product : Product  Inputs=3
  R1 : Constant  Value=0.5*1.225*3.14
  Radius : Constant  Value=77^5
  "lambda_opt " : Constant  Value=8.1
  K-opt : Outport
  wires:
  Divide/1 -> Product/1
  Radius/1 -> Product/2
  R1/1 -> Product/3
  Fcn/1 -> Divide/2
  "lambda_opt "/1 -> Fcn/1
  Cp_max/1 -> Divide/1
  Product/1 -> K-opt/1

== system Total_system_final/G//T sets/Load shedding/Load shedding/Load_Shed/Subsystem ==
  Load L2 : Inport
  Load M5 : Inport  Port=2
  Load M6 : Inport  Port=3
  Load L3 : Inport  Port=4
  Load M7 : Inport  Port=5
  Subsystem : Subsystem
  Subsystem1 : Subsystem
  CB_B4B5_stat : Outport
  CB_B1B4_stat : Outport  Port=2
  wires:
  Load L3/1 -> Subsystem/1(Load L3)
  Load M7/1 -> Subsystem/3(Load M7)
  Subsystem/1(CB_B4B5_stat) -> Subsystem1/5(In10), CB_B4B5_stat/1
  Load L2/1 -> Subsystem1/1(Load L2)
  Load M5/1 -> Subsystem1/3(Load M5)
  Load M6/1 -> Subsystem1/4(Load M6)
  Subsystem1/1(CB_B1B4_stat) -> CB_B1B4_stat/1
  [CB2_auto2] -> Subsystem1/2(In4), Subsystem/2(In5)

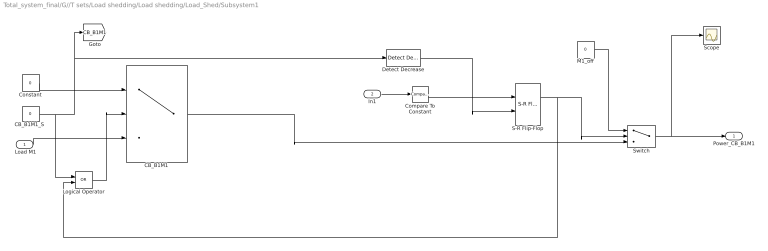
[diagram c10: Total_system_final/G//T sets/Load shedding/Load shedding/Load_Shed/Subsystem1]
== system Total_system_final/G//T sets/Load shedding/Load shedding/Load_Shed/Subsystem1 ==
  " Load M1" : Inport
  In1 : Inport  Port=2
  CB_B1M1 : Switch  Criteria=u2 ~= 0
  "CB_B1M1_S " : Constant  Value=0  OutDataTypeStr=boolean
  Compare To Constant : simulink/Logic and Bit Operations/Compare To Constant  relop===  const=10  OutDataTypeStr=boolean
  Constant : Constant  Value=0
  Detect Decrease : simulink/Logic and Bit Operations/Detect Decrease  vinit=0.0  OutDataTypeStr=boolean
  Logical Operator : Logic  Operator=OR  AllPortsSameDT=off  OutDataTypeStr=boolean
  M1_off : Constant  Value=0
  S-R Flip-Flop : simulink_extras/Flip Flops/S-R Flip-Flop  initial_condition=0
  Scope : Scope
  Switch : Switch  Threshold=0.24
  Power_CB_B1M1 : Outport
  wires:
  " Load M1"/1 -> CB_B1M1/3
  Constant/1 -> CB_B1M1/1
  "CB_B1M1_S "/1 -> Detect Decrease/1, [CB_B1M1], Logical Operator/1
  Compare To Constant/1 -> S-R Flip-Flop/1
  CB_B1M1/1 -> Switch/3
  S-R Flip-Flop/1 -> Logical Operator/2, Switch/2
  M1_off/1 -> Switch/1
  Switch/1 -> Scope/1, Power_CB_B1M1/1
  In1/1 -> Compare To Constant/1
  Detect Decrease/1 -> S-R Flip-Flop/2
  Logical Operator/1 -> CB_B1M1/2

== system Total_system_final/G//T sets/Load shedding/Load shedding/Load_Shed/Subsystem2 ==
  Load M2 : Inport
  In1 : Inport  Port=2
  CB_B1M2 : Switch  Criteria=u2 ~= 0
  "CB_B1M2_S  " : Constant  Value=0  OutDataTypeStr=boolean
  Compare To Constant1 : simulink/Logic and Bit Operations/Compare To Constant  relop===  const=11  OutDataTypeStr=boolean
  Constant1 : Constant  Value=0
  Constant2 : Constant  Value=0
  Detect Decrease : simulink/Logic and Bit Operations/Detect Decrease  vinit=0.0  OutDataTypeStr=boolean
  S-R Flip-Flop1 : simulink_extras/Flip Flops/S-R Flip-Flop  initial_condition=0
  Switch1 : Switch  Threshold=0.24
  Power_CB_B1M2 : Outport
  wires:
  "CB_B1M2_S  "/1 -> Detect Decrease/1, [CB_B1M2], CB_B1M2/2
  Load M2/1 -> CB_B1M2/3
  Constant1/1 -> CB_B1M2/1
  Switch1/1 -> Power_CB_B1M2/1
  S-R Flip-Flop1/1 -> Switch1/2
  Compare To Constant1/1 -> S-R Flip-Flop1/1
  CB_B1M2/1 -> Switch1/3
  In1/1 -> Compare To Constant1/1
  Constant2/1 -> Switch1/1
  Detect Decrease/1 -> S-R Flip-Flop1/2

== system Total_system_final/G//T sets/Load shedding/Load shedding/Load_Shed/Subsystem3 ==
  In1 : Inport
  Load L1 : Inport  Port=2
  CB_B1L1 : Switch  Criteria=u2 ~= 0
  CB_B1L1_S : Constant  Value=0  OutDataTypeStr=boolean
  Compare To Constant2 : simulink/Logic and Bit Operations/Compare To Constant  relop===  const=12  OutDataTypeStr=boolean
  Constant2 : Constant  Value=0
  Detect Decrease : simulink/Logic and Bit Operations/Detect Decrease  vinit=0.0  OutDataTypeStr=boolean
  S-R Flip-Flop2 : simulink_extras/Flip Flops/S-R Flip-Flop  initial_condition=0
  Switch2 : Switch  Threshold=0.24
  Power_CB_B1L1 : Outport
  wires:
  CB_B1L1/1 -> Switch2/3
  Compare To Constant2/1 -> S-R Flip-Flop2/1
  CB_B1L1_S/1 -> [CB_B1L1], Detect Decrease/1, CB_B1L1/2
  Load L1/1 -> CB_B1L1/3
  Constant2/1 -> CB_B1L1/1
  In1/1 -> Compare To Constant2/1
  S-R Flip-Flop2/1 -> Switch2/2
  Switch2/1 -> Power_CB_B1L1/1
  Detect Decrease/1 -> S-R Flip-Flop2/2

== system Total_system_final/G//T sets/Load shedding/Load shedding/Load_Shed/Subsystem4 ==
  Load M3 : Inport
  In5 : Inport  Port=2
  CB_B1M3 : Switch  Criteria=u2 ~= 0
  CB_B1M3_S : Constant  Value=0  OutDataTypeStr=boolean
  Compare To Constant6 : simulink/Logic and Bit Operations/Compare To Constant  relop===  const=14  OutDataTypeStr=boolean
  Constant1 : Constant  Value=0
  Constant3 : Constant  Value=0
  Detect Decrease : simulink/Logic and Bit Operations/Detect Decrease  vinit=0.0  OutDataTypeStr=boolean
  S-R Flip-Flop4 : simulink_extras/Flip Flops/S-R Flip-Flop  initial_condition=0
  Switch4 : Switch  Threshold=0.24
  Power_CB_B1M3 : Outport
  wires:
  In5/1 -> Compare To Constant6/1
  Load M3/1 -> CB_B1M3/3
  Constant3/1 -> CB_B1M3/1
  CB_B1M3_S/1 -> Detect Decrease/1, [CB_B1M3], CB_B1M3/2
  Compare To Constant6/1 -> S-R Flip-Flop4/1
  CB_B1M3/1 -> Switch4/3
  Switch4/1 -> Power_CB_B1M3/1
  S-R Flip-Flop4/1 -> Switch4/2
  Constant1/1 -> Switch4/1
  Detect Decrease/1 -> S-R Flip-Flop4/2

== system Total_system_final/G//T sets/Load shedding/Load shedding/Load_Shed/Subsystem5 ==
  In3 : Inport
  Load M4 : Inport  Port=2
  CB_B1M4 : Switch  Criteria=u2 ~= 0
  CB_B1M4_S : Constant  OutDataTypeStr=boolean
  Compare To Constant4 : simulink/Logic and Bit Operations/Compare To Constant  relop===  const=15  OutDataTypeStr=boolean
  Constant1 : Constant  Value=0
  Constant4 : Constant  Value=0
  Detect Decrease : simulink/Logic and Bit Operations/Detect Decrease  vinit=0.0  OutDataTypeStr=boolean
  S-R Flip-Flop5 : simulink_extras/Flip Flops/S-R Flip-Flop  initial_condition=0
  Switch5 : Switch  Criteria=u2 ~= 0  Threshold=0.24
  Power_CB_B1M4 : Outport
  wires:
  In3/1 -> Compare To Constant4/1
  Constant4/1 -> [CB_B1M4], CB_B1M4/1
  Load M4/1 -> CB_B1M4/3
  CB_B1M4_S/1 -> Detect Decrease/1, CB_B1M4/2
  CB_B1M4/1 -> Switch5/3
  Compare To Constant4/1 -> S-R Flip-Flop5/1
  S-R Flip-Flop5/1 -> Switch5/2
  Switch5/1 -> Power_CB_B1M4/1
  Constant1/1 -> Switch5/1
  Detect Decrease/1 -> S-R Flip-Flop5/2

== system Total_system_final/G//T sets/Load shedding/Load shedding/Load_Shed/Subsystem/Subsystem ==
  Load L3 : Inport
  In5 : Inport  Port=2
  Load M7 : Inport  Port=3
  Add1 : Sum
  CB_B4B5 : Switch  Criteria=u2 ~= 0
  CB_B4B5_S : Constant  Value=0  OutDataTypeStr=boolean
  Compare To Constant5 : simulink/Logic and Bit Operations/Compare To Constant  relop===  const=16  OutDataTypeStr=boolean
  Constant1 : Constant  Value=0
  Constant2 : Constant  Value=0
  Detect Decrease : simulink/Logic and Bit Operations/Detect Decrease  vinit=0.0  OutDataTypeStr=boolean
  S-R Flip-Flop6 : simulink_extras/Flip Flops/S-R Flip-Flop  initial_condition=0
  Switch6 : Switch  Threshold=0.24
  CB_B4B5_stat : Outport
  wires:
  In5/1 -> Compare To Constant5/1
  Load M7/1 -> Add1/2
  Load L3/1 -> Add1/1
  Add1/1 -> CB_B4B5/3
  Constant1/1 -> CB_B4B5/1
  CB_B4B5_S/1 -> Detect Decrease/1, [CB_B4B5], CB_B4B5/2
  CB_B4B5/1 -> Switch6/3
  Switch6/1 -> CB_B4B5_stat/1
  S-R Flip-Flop6/1 -> Switch6/2
  Compare To Constant5/1 -> S-R Flip-Flop6/1
  Constant2/1 -> Switch6/1
  Detect Decrease/1 -> S-R Flip-Flop6/2

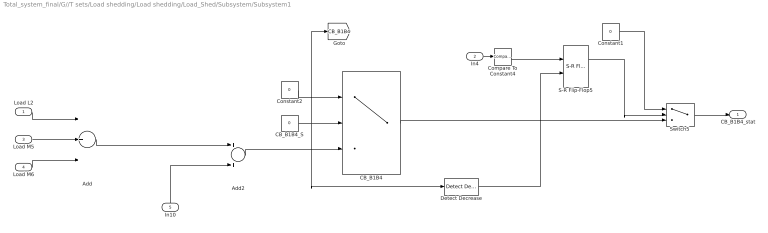
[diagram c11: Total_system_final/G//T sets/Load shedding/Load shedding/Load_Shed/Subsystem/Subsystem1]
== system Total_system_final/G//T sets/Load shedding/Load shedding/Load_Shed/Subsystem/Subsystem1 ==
  Load L2 : Inport
  In4 : Inport  Port=2
  Load M5 : Inport  Port=3
  Load M6 : Inport  Port=4
  In10 : Inport  Port=5
  Add : Sum  Inputs=+++
  Add2 : Sum
  CB_B1B4 : Switch  Criteria=u2 ~= 0
  CB_B1B4_S : Constant  Value=0  OutDataTypeStr=boolean
  Compare To Constant4 : simulink/Logic and Bit Operations/Compare To Constant  relop===  const=15  OutDataTypeStr=boolean
  Constant1 : Constant  Value=0
  Constant2 : Constant  Value=0
  Detect Decrease : simulink/Logic and Bit Operations/Detect Decrease  vinit=0.0  OutDataTypeStr=boolean
  S-R Flip-Flop5 : simulink_extras/Flip Flops/S-R Flip-Flop  initial_condition=0
  Switch5 : Switch  Threshold=0.24
  CB_B1B4_stat : Outport
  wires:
  In4/1 -> Compare To Constant4/1
  Load L2/1 -> Add/1
  Load M6/1 -> Add/3
  Load M5/1 -> Add/2
  Add/1 -> Add2/1
  Add2/1 -> CB_B1B4/3
  Constant2/1 -> CB_B1B4/1
  CB_B1B4_S/1 -> Detect Decrease/1, [CB_B1B4], CB_B1B4/2
  In10/1 -> Add2/2
  Switch5/1 -> CB_B1B4_stat/1
  CB_B1B4/1 -> Switch5/3
  S-R Flip-Flop5/1 -> Switch5/2
  Compare To Constant4/1 -> S-R Flip-Flop5/1
  Constant1/1 -> Switch5/1
  Detect Decrease/1 -> S-R Flip-Flop5/2

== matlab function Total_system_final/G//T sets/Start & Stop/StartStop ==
function [wset1, wset2, CB_auto]  = start_stop(P_Gen, CB_man, w1, w2, start_stop_G1 , start_stop_G2, auto, Connect) 


droop = 0.04;

if start_stop_G1 == 1
    
    wset1 = 1;

else 
    
    wset1 = 0;

end



if (start_stop_G2 == 1) & (CB_man == 0) & (Connect == 0)
    
    wset2 = w1;
    
elseif  (start_stop_G2 == 1) & (CB_man == 1) & (Connect == 0)
     
    wset2 = 1; 
    
elseif (w1 ~= w2) & (start_stop_G1 == 1) & (start_stop_G2 == 1) & (Connect == 1)
    
    wset2 = w1+(P_Gen*droop/2);
    
else
    
    wset2 = 0;

end
    



% if start_stop_G2 == 1 & (CB_man == 1)
%     
%     wset2 = 1;  
%     
% else  
%     
%     wset2 = 0;
% 
% end


if (w1 ~= w2) & (start_stop_G1 == 1) & (start_stop_G2 == 1) & (auto == 1)
    
 
   CB_auto = 1;
 
else 
     
   CB_auto = 0;
    
end
    
    
%     
% if (w1 ~= w2) & (start_stop_G1 == 1) & (start_stop_G2 == 1) & (CB_man == 1)
%       
%   
%      wset2 = 1; % wset2 = w1+(P_G1*droop/2);
%   
% else 
%       
%    
%     
% end

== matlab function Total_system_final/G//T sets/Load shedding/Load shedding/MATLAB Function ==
function [CB_B1M1_stat, CB_B1M2_stat, CB_B1L1_stat, CB_B1M3_stat, CB_B1M4_stat ,CB_B1B4_stat, CB_B4B5_stat, idx] = LoadShed(freq, CB_B1M1, CB_B1M2, CB_B1L1, CB_B1M3, CB_B1M4,CB_B1B4, CB_B4B5, P_CB_B1M1, P_CB_B1M2, P_CB_B1L1, P_CB_B1M3, P_CB_B1M4, P_CB_B1B4, P_CB_B4B5)

%Initial conditions

CB_B1M1_stat = 0;
CB_B1M2_stat = 0;
CB_B1L1_stat = 0;
CB_B1M3_stat = 0;
CB_B1M4_stat = 0;
CB_B1B4_stat = 0;
CB_B4B5_stat = 0;


Power = [P_CB_B1M1 P_CB_B1M2 P_CB_B1L1 P_CB_B1M3 P_CB_B1M4 P_CB_B1B4 P_CB_B4B5];

droop = 0.04;

freq_limit = 0.98;

delta_freq = freq_limit - freq;

P_shed = delta_freq/droop;

[~,idx] = min(abs(Power-P_shed));

% [~,idx] = min(abs(Power-P_overload));
    
if (freq < freq_limit & idx == 1 & CB_B1M1 == 0)
    
    CB_B1M1_stat = 1;
    
elseif (freq < freq_limit & idx == 2 & CB_B1M2 == 0)
    
    CB_B1M2_stat = 1; 

elseif (freq < freq_limit & idx == 3 & CB_B1L1 == 0)
    
    CB_B1L1_stat = 1;
    
elseif (freq < freq_limit & idx == 4 & CB_B1M3 == 0)
    
    CB_B1M3_stat = 1;    


elseif (freq < freq_limit & idx == 5 & CB_B1M4 == 0)
    
    CB_B1M4_stat = 1;
    

elseif (freq < freq_limit & idx == 6 & CB_B1B4 == 0)
    
    CB_B1B4_stat = 1;
    

elseif (freq < freq_limit & idx == 7 & CB_B4B5 == 0)
    
    CB_B4B5_stat = 1;
    

else
    
    
end

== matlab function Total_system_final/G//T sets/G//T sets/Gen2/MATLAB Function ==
function x  = speed(w1,w2,CB)


if ((w1 - w2) > 0.05) | (CB == 0)
    
    x = 1;
    
else
    
    x = 0;

end

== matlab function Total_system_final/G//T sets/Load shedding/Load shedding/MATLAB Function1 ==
function [Power,idx2, CB] = fcn(P_load, P_wind, P_CB_B1M1, P_CB_B1M2, P_CB_B1L1, P_CB_B1M3, P_CB_B1M4, P_CB_B1B4, P_CB_B4B5)


%Initial conditions

CB = 0;

Power = [P_CB_B1M1 P_CB_B1M2 P_CB_B1L1 P_CB_B1M3 P_CB_B1M4 P_CB_B1B4 P_CB_B4B5];


%Automatic loadsheddig if overload

P_shed = P_load - P_wind - 1;

[~,idx2] = min(abs(P_shed + 0.05));



if (P_shed > 0 & idx2 == 1)
    
    CB = 1;
    
elseif (P_shed > 0 & idx2 == 2)
    
    CB = 2; 

elseif (P_shed > 0 & idx2 == 3)
    
    CB = 3;
    
elseif (P_shed > 0 & idx2 == 4)
    
    CB = 4;    

elseif (P_shed > 0 & idx2 == 5)
    
    CB = 5;

elseif (P_shed > 0 & idx2 == 6)
    
    CB = 6;

elseif (P_shed > 0 & idx2 == 7)
    
    CB = 7;

else
    

    
end
